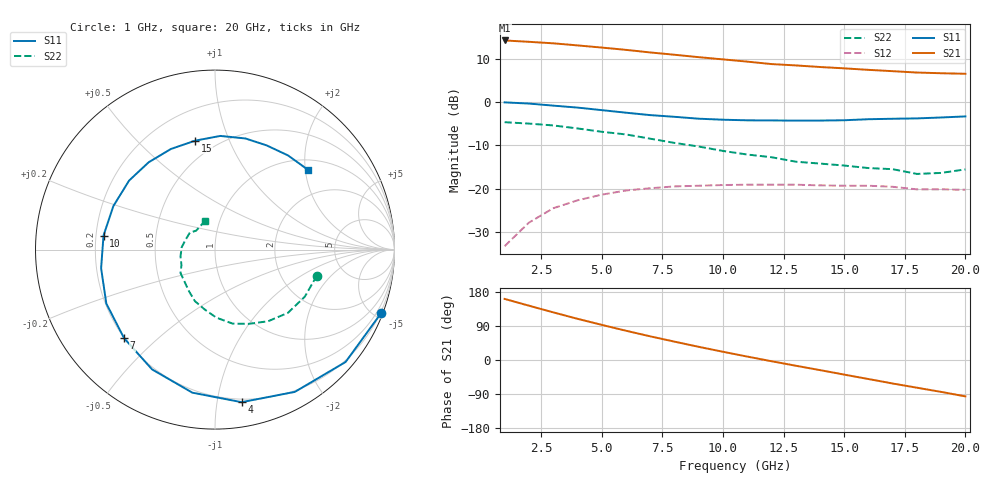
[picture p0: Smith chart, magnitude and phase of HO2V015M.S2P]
! SIEMENS Small Signal Semiconductors
! CFY67-10
! GaAs HEMT in Micro-X
! VDS = 2 V  ID = 15 mA
! Common Source S-Parameters:  August 1993
# GHz  S  MA  R  50
!  f  S11  S21  S12  S22
! GHz  MAG  ANG  MAG  ANG  MAG  ANG  MAG  ANG
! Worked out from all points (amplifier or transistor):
!   20 points, 1 GHz to 20 GHz, reference 50 ohm
!   highest |S21| = 14.2 dB at 1 GHz (marker M1)
!   |S21| within 3 dB of that: start of sweep to 7.465 GHz
!   unconditionally stable (mu >= 1): 12.12 GHz to end of sweep
!   at 4 GHz: K = 0.37, MSG = 17.8 dB, |S12| = -22.6 dB
!   at 11 GHz: K = 0.94, MSG = 14.2 dB, |S12| = -19.0 dB
!   at 20 GHz: K = 1.26, MAG = 10.3 dB, |S12| = -20.2 dB
!   lowest NFmin = 0.39 dB at 2 GHz
!   S11 on the Smith chart (normalised r, x): 1 GHz: 0.14, -5.42; 4 GHz: 0.18, -1.17; 7 GHz: 0.20, -0.39; 10 GHz: 0.23, +0.06; 15 GHz: 0.39, +0.76; 20 GHz: 1.25, +2.07
1  0.991 -20.9  5.103 161.2  0.022 76.6  0.586 -14.3
2  0.96 -40.7  4.923 143.4  0.041 63.6  0.565 -27.6
3  0.909 -60.7  4.732 125.8  0.06 50.6  0.538 -40.9
4  0.863 -80.1  4.479 108.8  0.074 39.1  0.497 -53.4
5  0.807 -99.0  4.229 92.8  0.086 28.3  0.455 -65.4
6  0.754 -117.7  3.979 77.3  0.096 17.5  0.424 -76.6
7  0.707 -135.8  3.717 62.5  0.102 8.0  0.379 -88.9
8  0.676 -153.6  3.496 48.5  0.107 -0.6  0.339 -99.6
9  0.643 -170.7  3.279 34.8  0.109 -9.1  0.308 -111.4
10  0.626 172.8  3.091 21.8  0.111 -17.0  0.274 -121.8
11  0.616 156.8  2.915 9.1  0.112 -24.3  0.249 -132.1
12  0.614 141.2  2.731 -3.2  0.112 -31.2  0.232 -146.0
13  0.611 127.2  2.636 -15.0  0.112 -38.4  0.206 -155.1
14  0.612 113.7  2.527 -26.6  0.11 -44.8  0.196 -168.8
15  0.617 100.3  2.439 -38.5  0.109 -51.4  0.186 175.9
16  0.634 87.3  2.343 -50.2  0.109 -58.6  0.174 163.3
17  0.642 74.7  2.263 -62.0  0.106 -65.7  0.169 146.1
18  0.648 63.6  2.182 -73.1  0.099 -72.3  0.149 135.0
19  0.664 52.2  2.142 -84.2  0.099 -77.3  0.153 124.2
20  0.683 40.5  2.112 -96.0  0.098 -85.1  0.168 109.5
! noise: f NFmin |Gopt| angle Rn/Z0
2  0.39  0.79  27  0.28
4  0.52  0.74  55  0.22
6  0.61  0.68  85  0.15
8  0.71  0.62  117  0.08
10  0.81  0.57  149  0.04
12  0.9  0.54  -177  0.02
14  1.01  0.52  -144  0.05
16  1.11  0.51  -112  0.12
18  1.22  0.51  -84  0.22
20  1.31  0.51  -56  0.33
